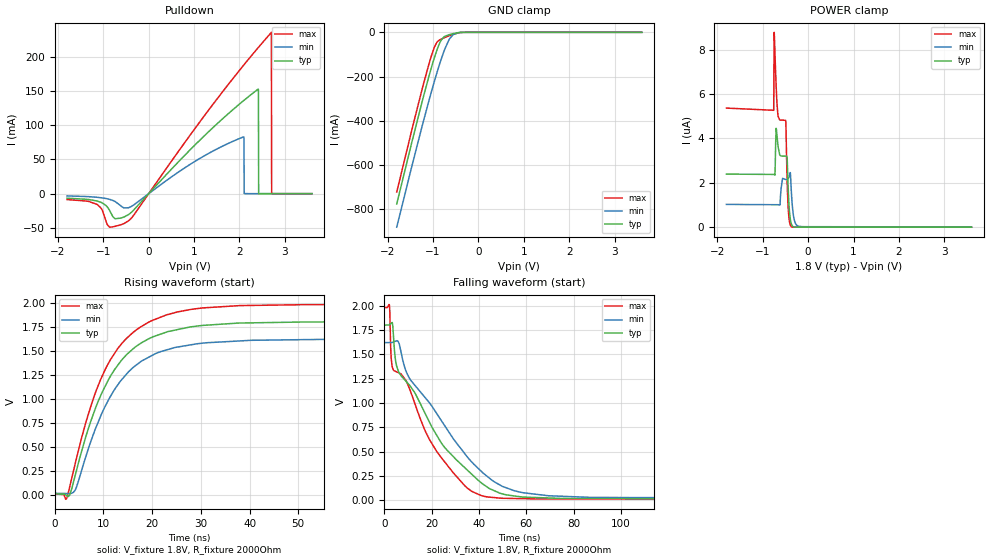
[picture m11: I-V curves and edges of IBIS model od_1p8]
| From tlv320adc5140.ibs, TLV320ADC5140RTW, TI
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|   od_1p8 Model
[Model]   od_1p8
Model_type   I/O_open_drain
Polarity   Non-Inverting
Enable   Active-Low
Vinl = 0.54
Vinh = 1.26
Vmeas = 0.9
Vref = 1.8
Cref = 2pF
Rref = 2000
|   typ   min   max
C_comp   1.913pF   1.861pF   1.994pF
[Model spec]
|subparameter
Vinl   0.54   0.486   0.594
Vinh   1.26   1.134   1.386
| Where Nom  PVT is Nominal Process, 1.8V, 27C
|   Fast PVT is Strong Process,  1.98V, -40C
|   Slow PVT is Weak Process,   1.62V, 150C
[Voltage Range]   1.8   1.62   1.98
|Junction Temperature
[Temperature Range]   27   150   -40
[Pullup Reference]   1.8   1.62   1.98
[Pulldown Reference]   0   0   0
[Power Clamp Reference]   1.8   1.62   1.98
[GND Clamp Reference]   0   0   0
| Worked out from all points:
|   slope of the pulldown table from 0 to 0.27 V, typ, clamps not added: 13.9 ohm
|   GND clamp passes 1 mA (typ) near -0.42 V on its own axis
|   falling waveform, V_fixture 1.8V, R_fixture 2000Ohm: 20-80 % time 27.8ns typ, 29.6ns min, 22.5ns max; typ from 1.8 V to 0.013 V
|   rising waveform, V_fixture 1.8V, R_fixture 2000Ohm: 20-80 % time 9.4ns typ, 9.53ns min, 9.4ns max; typ from 0.013 V to 1.8 V
[Pulldown]
|   Voltage   I(typ)   I(min)   I(max)
-1.8V     -6.578mA   -3.262mA   -8.574mA
-865.8mV  -23.95mA   -8.274mA   -48.75mA
-444.6mV  -30.6mA    -20.56mA   -39.64mA
2.093V    135.8mA    82.85mA    187.5mA
2.099V    136.1mA    80.63mA    187.9mA
2.104V    136.4mA    382.3uA    188.4mA
2.412V    152.6mA    169.6nA    212.9mA
2.417V    151.5mA    168.5nA    213.4mA
2.423V    25.41nA    167.3nA    213.8mA
2.704V    1.52nA     125nA      235.3mA
2.709V    2.184nA    124.4nA    -21.3nA
3.6V      908pA      71.03nA    80.42pA
[GND Clamp]
|   Voltage   I(typ)   I(min)   I(max)
-1.8V     -775mA     -880mA     -721.6mA
-1.249V   -320.2mA   -430.6mA   -263.5mA
-1.087V   -196.1mA   -306.3mA   -140.9mA
-979.2mV  -120.4mA   -227.5mA   -72.1mA
-909mV    -76.89mA   -178.8mA   -43.52mA
-828mV    -37.7mA    -126.1mA   -31.51mA
-763.2mV  -20.89mA   -87.78mA   -25.59mA
-649.8mV  -10.89mA   -34.03mA   -15.87mA
-558mV    -5.899mA   -10.52mA   -9.077mA
-444.6mV  -1.487mA   -2.035mA   -2.625mA
-298.8mV  -23.62uA   -99.24uA   -23.6uA
3.6V      0A         0A         0A
[POWER Clamp]
|   Voltage   I(typ)   I(min)   I(max)
-1.8V     2.389uA    1.025uA    5.362uA
-757.8mV  2.375uA    1.011uA    5.264uA
-747mV    2.374uA    1.011uA    8.776uA
-730.8mV  2.342uA    1.011uA    7.826uA
-703.8mV  4.452uA    1.011uA    6.313uA
-660.6mV  3.605uA    1.011uA    4.99uA
-493.2mV  3.202uA    2.144uA    4.807uA
-466.2mV  3.188uA    2.151uA    2.367uA
-428.4mV  1.247uA    2.224uA    548.1nA
-374.4mV  180.3nA    1.777uA    32.15nA
-217.8mV  0A         45.37nA    0A
3.6V      0A         0A         0A
[Ramp]
R_load = 2000
|   typ   min   max
dV/dt_r   1.07232/9.40454e-09   0.961564/9.53433e-09   1.1817/9.39999e-09
dV/dt_f   1.07232/2.77178e-08   0.961564/2.9589e-08   1.1817/2.25157e-08
[Falling Waveform]
V_fixture = 1.8V
V_fixture_min = 1.62V
V_fixture_max = 1.98V
R_fixture = 2000Ohm
C_fixture = 0F
|   Time   V(typ)   V(min)   V(max)
0s        1.8V       1.62V      1.98V
2.116ns   1.805V     1.621V     2.003V
2.784ns   1.818V     1.621V     1.485V
3.705ns   1.725V     1.626V     1.343V
6.159ns   1.313V     1.61V      1.308V
10.61ns   1.183V     1.252V     1.145V
22.1ns    668.7mV    891.4mV    502.7mV
40.95ns   179.8mV    297.8mV    48.68mV
69.32ns   24.58mV    47.34mV    13.7mV
250ns     12.8mV     17.33mV    10.51mV
[Rising Waveform]
V_fixture = 1.8V
V_fixture_min = 1.62V
V_fixture_max = 1.98V
R_fixture = 2000Ohm
C_fixture = 0F
|   Time   V(typ)   V(min)   V(max)
0s        12.8mV     17.33mV    10.51mV
2.431ns   -4.221mV   15.13mV    -38.03mV
3.093ns   3.627mV    14.53mV    90.43mV
4.299ns   224.4mV    62.46mV    348.3mV
7.664ns   804.8mV    593.4mV    964.2mV
10.34ns   1.13V      920.7mV    1.303V
12.88ns   1.345V     1.141V     1.518V
17.79ns   1.581V     1.391V     1.752V
27.89ns   1.747V     1.561V     1.928V
250ns     1.8V       1.62V      1.98V
